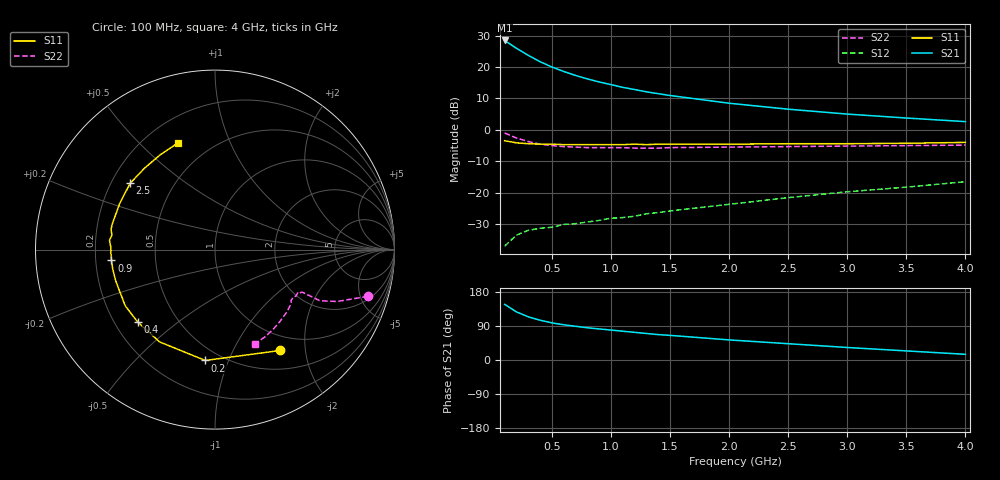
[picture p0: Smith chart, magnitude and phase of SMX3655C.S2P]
! HSMX-3655 Common Emitter
! Vce=10V Ic=15ma
# ghz s ma r 50
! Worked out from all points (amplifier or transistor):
!   20 points, 100 MHz to 4 GHz, reference 50 ohm
!   highest |S21| = 28.5 dB at 100 MHz (marker M1)
!   |S21| within 3 dB of that: start of sweep to 223 MHz
!   unconditionally stable (mu >= 1): 986.4 MHz to 3.026 GHz
!   at 400 MHz: K = 0.57, MSG = 26.5 dB, |S12| = -31.4 dB
!   at 1.1 GHz: K = 1.09, MAG = 18.9 dB, |S12| = -28.0 dB
!   at 4 GHz: K = 0.83, MSG = 9.6 dB, |S12| = -16.5 dB
!   S11 on the Smith chart (normalised r, x): 100 MHz: 0.77, -1.56; 200 MHz: 0.41, -0.83; 400 MHz: 0.29, -0.36; 900 MHz: 0.27, -0.05; 2.5 GHz: 0.28, +0.32; 4 GHz: 0.33, +0.66
0.1  0.67 -57.0  26.5 147.0  0.014 62.0  0.89 -17.0
0.2  0.62 -95.0  19.92 127.0  0.021 51.0  0.74 -23.0
0.3  0.6 -121.0  15.35 114.0  0.025 47.0  0.65 -26.0
0.4  0.59 -137.0  12.17 105.0  0.027 46.0  0.59 -26.0
0.5  0.59 -148.0  10 98.0  0.028 46.0  0.56 -26.0
0.6  0.58 -156.0  8.5 93.0  0.031 47.0  0.54 -26.0
0.7  0.58 -163.0  7.35 89.0  0.032 49.0  0.53 -27.0
0.8  0.58 -169.0  6.48 85.0  0.034 52.0  0.52 -27.0
0.9  0.58 -174.0  5.78 82.0  0.036 52.0  0.52 -28.0
1  0.58 -178.0  5.25 79.0  0.039 54.0  0.52 -29.0
1.1  0.58 179.0  4.74 76.0  0.04 53.0  0.52 -30.0
1.2  0.59 175.0  4.38 73.0  0.042 57.0  0.51 -31.0
1.3  0.58 172.0  4.03 70.0  0.046 58.0  0.51 -33.0
1.4  0.59 169.0  3.76 67.0  0.048 59.0  0.51 -34.0
1.5  0.59 166.0  3.52 65.0  0.051 62.0  0.52 -35.0
2  0.59 154.0  2.65 53.0  0.065 66.0  0.53 -41.0
2.5  0.6 142.0  2.13 43.0  0.083 68.0  0.54 -48.0
3  0.6 131.0  1.78 33.0  0.103 66.0  0.55 -54.0
3.5  0.61 120.0  1.54 24.0  0.122 66.0  0.56 -60.0
4  0.63 109.0  1.35 15.0  0.149 64.0  0.57 -67.0
